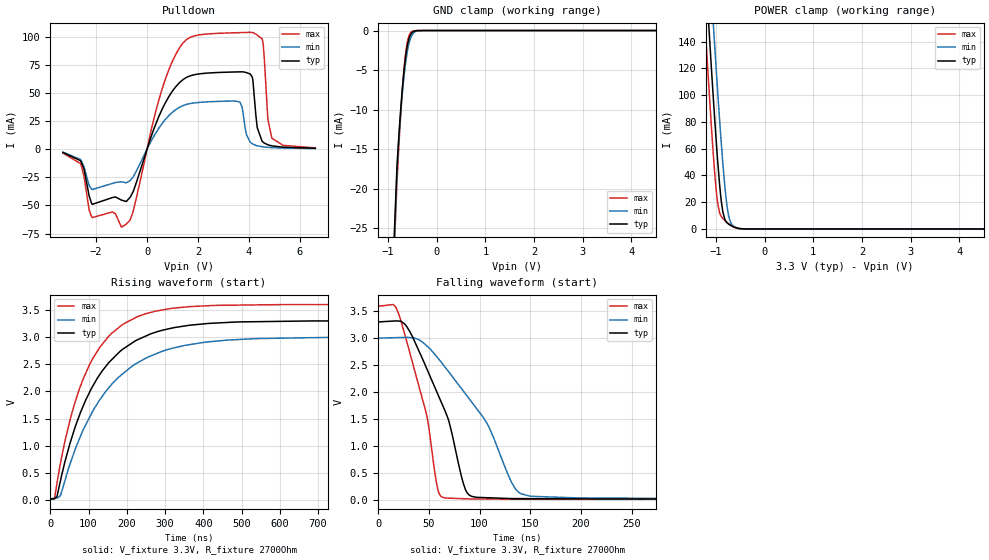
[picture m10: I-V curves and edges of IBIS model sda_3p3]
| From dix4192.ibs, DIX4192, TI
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|   sda_3p3 Model
[Model]   sda_3p3
Model_type   I/O_open_drain
Polarity   Non-Inverting
Enable   Active-Low
Vinl = 0.99
Vinh = 2.31
Vmeas = 1.65
Vref = 3.3
Cref = 2pF
Rref = 2000
|   typ   min   max
C_comp   31.7425pF   25.9202pF   37.4662pF
|C_comp_pulldown   31.8889pF   26.04pF   37.8106pF
[Model spec]
|subparameter
Vinl   0.99   0.90   1.08
Vinh   2.31   2.10   2.52
| Where nom  PVT is Nominal Process, 3.3V, 27C
|   Fast PVT is Strong Process,  3.6V, -40C
|   Slow PVT is Weak Process,   3.0V, 105C
[Voltage Range]   3.3   3   3.6
[Temperature Range]   27   105   -40
[Pullup Reference]   3.3   3   3.6
[Pulldown Reference]   0   0   0
[Power Clamp Reference]   3.3   3   3.6
[GND Clamp Reference]   0   0   0
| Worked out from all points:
|   slope of the pulldown table from 0 to 0.495 V, typ, clamps not added: 16.2 ohm
|   GND clamp passes 1 mA (typ) near -0.56 V on its own axis
|   POWER clamp passes 1 mA (typ) near -0.59 V on its own axis
|   falling waveform, V_fixture 3.3V, R_fixture 2700Ohm: 20-80 % time 36.1ns typ, 56.5ns min, 25.2ns max; typ from 3.3 V to 0.017 V
|   rising waveform, V_fixture 3.3V, R_fixture 2700Ohm: 20-80 % time 132ns typ, 154ns min, 109ns max; typ from 0.017 V to 3.3 V
[Pulldown]
|   Voltage   I(typ)   I(min)   I(max)
-3.3V     -2.999mA   -2.604mA   -3.4mA
-2.607V   -10.48mA   -9.369mA   -13.22mA
-2.171V   -48.36mA   -35.62mA   -60.29mA
-815.1mV  -46.48mA   -29.91mA   -66.62mA
551.1mV   33.46mA    21.47mA    50.4mA
1.284V    59.26mA    37.28mA    90.3mA
3.62V     68.62mA    41.95mA    103.4mA
4.036V    66.86mA    6.565mA    103.7mA
4.541V    6.437mA    2.072mA    95.45mA
4.739V    3.875mA    1.619mA    26.56mA
4.897V    2.922mA    1.376mA    9.736mA
6.6V      785.7uA    521.4uA    1.132mA
[GND Clamp]
|   Voltage   I(typ)   I(min)   I(max)
-3.3V     -1.052A    -978.4mA   -1.121A
-1.003V   -46.85mA   -48.77mA   -48.16mA
-815.1mV  -17.3mA    -17.98mA   -19.31mA
-765.6mV  -12.4mA    -12.84mA   -13.54mA
-716.1mV  -8.26mA    -8.79mA    -8.564mA
-676.5mV  -5.518mA   -6.188mA   -5.319mA
-636.9mV  -3.351mA   -4.098mA   -2.883mA
-577.5mV  -1.26mA    -1.896mA   -834.3uA
-528mV    -443.2uA   -845.6uA   -222.7uA
-478.5mV  -130.9uA   -327.2uA   -47.39uA
-260.7mV  0A         -1.313uA   0A
6.6V      0A         0A         0A
[POWER Clamp]
|   Voltage   I(typ)   I(min)   I(max)
-3.3V     1.547A     1.6A       1.506A
-1.261V   221.8mA    278.9mA    176.5mA
-1.201V   185.4mA    242.4mA    140.3mA
-1.181V   173.4mA    230.3mA    128.4mA
-1.092V   120.7mA    176.8mA    76.94mA
-1.063V   103.7mA    159.3mA    60.97mA
-1.033V   87.14mA    142.1mA    46.08mA
-963.6mV  51.24mA    103.1mA    19.41mA
-854.7mV  12.41mA    48.08mA    7.805mA
-745.8mV  3.823mA    11.52mA    4.15mA
-607.2mV  1.171mA    1.445mA    1.051mA
6.6V      0A         0A         0A
[Ramp]
R_load = 2700
|   typ   min   max
dV/dt_r   1.96988/1.30737e-07   1.78574/1.52852e-07   2.15265/1.08772e-07
dV/dt_f   1.96988/3.61061e-08   1.78574/5.64647e-08   2.15265/2.52396e-08
[Falling Waveform]
V_fixture = 3.3V
V_fixture_min = 3V
V_fixture_max = 3.6V
R_fixture = 2700Ohm
C_fixture = 0F
|   Time   V(typ)   V(min)   V(max)
0s        3.3V       3V         3.6V
20.07ns   3.317V     3.01V      3.457V
48.12ns   2.425V     2.854V     1.547V
58.68ns   1.966V     2.635V     206.5mV
65.69ns   1.661V     2.468V     39.45mV
89.79ns   92.05mV    1.875V     19.46mV
108.6ns   41.34mV    1.375V     17.1mV
135ns     25.88mV    216.6mV    15.11mV
150.8ns   24.47mV    70.41mV    13.91mV
1.25us    16.86mV    23.73mV    12.26mV
[Rising Waveform]
V_fixture = 3.3V
V_fixture_min = 3V
V_fixture_max = 3.6V
R_fixture = 2700Ohm
C_fixture = 0F
|   Time   V(typ)   V(min)   V(max)
0s        16.86mV    23.73mV    12.26mV
11.37ns   23.39mV    32.02mV    42.44mV
27.13ns   371.7mV    90.58mV    696.4mV
63.67ns   1.314V     905.2mV    1.777V
101.1ns   1.962V     1.501V     2.469V
152.5ns   2.526V     2.063V     3.014V
225.8ns   2.944V     2.518V     3.37V
321.9ns   3.172V     2.799V     3.533V
461.9ns   3.269V     2.944V     3.586V
1.25us    3.3V       3V         3.6V
